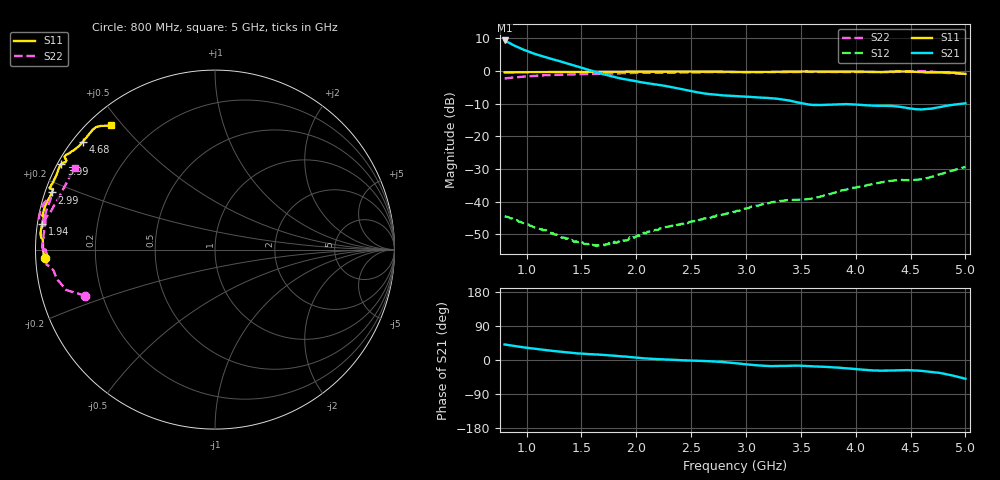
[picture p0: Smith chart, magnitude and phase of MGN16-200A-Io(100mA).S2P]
! Port[1] = GATE
! Port[2] = DRAIN
! [Type]  S-parameter s2p file
! [Object]  MGN16-200A
! [Bias]  100 mA
! [Version]  1.0
! [Date]  Jul 2026
! [Source]  This file was created in JSC "ICC Milandr".
! [Disclaimer] Property of JSC "ICC Milandr". Unauthorized reproduction and/or distribution is strictly prohibited.
!  The file and the data are provided "AS IS" and with all faults and disclaim all warranties, express and implied, including
!  without limitation any implied warranties of merchantability, fitness for a particular purpose.
!  JSC "ICC Milandr" assumes no liability for:
!  1) the accuracy of the data provided;
!  2) the proper functioning of this data;
!  3) infringement of patents, copyrights or intellectual property rights resulting from the use of this data.
!  JSC "ICC Milandr" reserves the right to make changes to the products and the data without prior notice.
!  Please, be aware that your receipt and use of the file provided shall serve as acceptance of these terms and conditions.
!  If you do not accept these terms, you should return or destroy this file and any other accompanying information immediately.
# GHZ S MA R 50
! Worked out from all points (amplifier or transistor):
!   421 points, 800 MHz to 5 GHz, reference 50 ohm
!   highest |S21| = 9.3 dB at 800 MHz (marker M1)
!   |S21| within 3 dB of that: start of sweep to 985.2 MHz
!   unconditionally stable (mu >= 1): 1.194 GHz to 2.064 GHz; 2.075 GHz to 2.134 GHz; 4.948 GHz to end of sweep
!   at 1.5 GHz: K = 1.25, MAG = 23.8 dB, |S12| = -52.7 dB
!   at 2.9 GHz: K = 0.62, MSG = 17.7 dB, |S12| = -43.2 dB
!   at 5 GHz: K = 1.18, MAG = 7.2 dB, |S12| = -29.3 dB
!   S11 on the Smith chart (normalised r, x): 800 MHz: 0.03, -0.03; 1.94 GHz: 0.01, +0.07; 2.99 GHz: 0.02, +0.17; 3.99 GHz: 0.01, +0.26; 4.68 GHz: 0.03, +0.36; 5 GHz: 0.06, +0.47
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0.8  0.9504 -177.1  2.932 41.0  0.006007 -30.5  0.7676 -160.3
0.89  0.9548 -178.4  2.441 36.9  0.005265 -31.6  0.7969 -162.0
0.94  0.9561 -179.2  2.237 34.8  0.004925 -31.3  0.8113 -162.7
1.08  0.9588 178.3  1.813 29.3  0.003986 -31.8  0.8452 -164.2
1.23  0.9612 176.8  1.529 24.1  0.003234 -28.4  0.8662 -165.7
1.5  0.971 176.1  1.121 16.7  0.002325 -3.9  0.8982 -170.3
1.66  0.9736 175.5  0.931 14.1  0.00214 17.4  0.9074 -172.6
1.94  0.9729 171.7  0.7248 7.9  0.002841 47.0  0.9317 -174.5
2.2  0.9737 169.0  0.614 2.2  0.0037 55.5  0.9386 -177.2
2.39  0.9805 168.9  0.5393 -0.2  0.004482 60.2  0.9453 180.0
2.6  0.9792 167.7  0.4575 -2.6  0.005335 65.1  0.9589 -179.5
2.9  0.9664 162.4  0.4135 -8.2  0.006952 65.7  0.9622 179.3
2.99  0.9625 160.7  0.4038 -11.1  0.007845 64.3  0.9618 178.3
3.38  0.9807 159.7  0.3567 -15.4  0.01051 65.3  0.9589 170.1
3.6  0.9795 158.3  0.3031 -16.6  0.01118 66.2  0.9704 171.2
3.77  0.9761 155.0  0.3048 -18.9  0.01314 65.4  0.9649 172.0
3.99  0.9798 150.8  0.3072 -23.7  0.01639 62.3  0.9642 169.2
4.3  0.9747 148.8  0.2927 -27.9  0.02062 55.9  0.9583 162.6
4.49  0.9817 147.3  0.2676 -26.9  0.02142 55.8  0.992 166.3
4.68  0.9503 140.7  0.2637 -31.1  0.02358 50.4  0.9809 170.8
4.81  0.9535 135.2  0.2908 -36.5  0.02756 44.9  0.9369 166.5
5  0.9016 129.8  0.3201 -49.3  0.03418 32.4  0.9058 149.7
